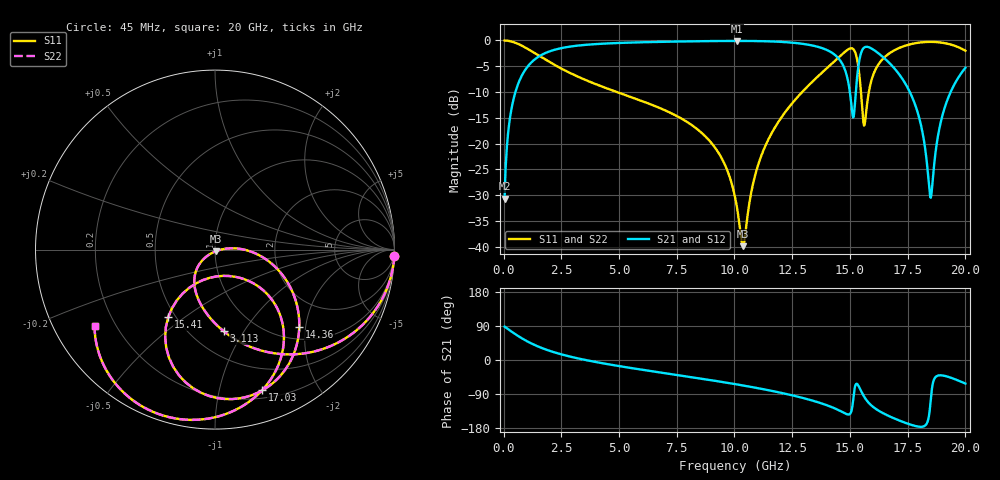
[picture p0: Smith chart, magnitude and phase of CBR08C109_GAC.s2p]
! S-parameter model data by Modelithics Inc.  support@modelithics.com 813-866-6335  Tampa FL USA
! S-Parameter data specifications:
! Substrate: 20-mil Rogers 4350B, substrate thickness, H=0.508mm, Dielectric constant, Er=3.75
! PCB Mounting Pad Footprint: Pad width, PadW=1.45mm , Pad length, PadL=1mm , Pad gap, PadG (edge-to-edge)=0.6mm , Reference planes=2.6mm apart
#  GHz  S  MA  R 50
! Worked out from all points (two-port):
!   801 points, 45 MHz to 20 GHz, reference 50 ohm
!   highest |S21| = -0.10 dB at 10.1 GHz (marker M1); lowest = -30.7 dB at 45 MHz (marker M2)
!   |S21| within 3 dB of the highest: 1.531 GHz to 14.42 GHz (12.89 GHz wide, 162 % of centre); 15.44 GHz to 16.4 GHz (958.7 MHz wide, 6.02 % of centre)
!   lowest |S11| = -39.9 dB at 10.37 GHz (marker M3), VSWR 1.02, Z = 50.4 - j0.946 ohm
!   |S11| at or under -10 dB: 4.911 GHz to 12.93 GHz (8.019 GHz wide, 89.9 % of centre); 15.48 GHz to 15.82 GHz (340.9 MHz wide, 2.18 % of centre)
!   |S22| runs from -39.9 to 0.0 dB; largest |S21 - S12| = 0
!   S11 on the Smith chart (normalised r, x): 45 MHz: 1, -58; 3.113 GHz: 0.71, -0.82; 14.36 GHz: 1.27, -1.85; 15.41 GHz: 0.46, -0.44; 17.03 GHz: 0.27, -1.35; 20 GHz: 0.12, -0.29
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0.045  0.9996 -2.0  0.02928 88.0  0.02928 88.0  0.9996 -2.0
0.319381  0.979 -14.0  0.2034 76.0  0.2034 76.0  0.979 -14.0
0.793312  0.8887 -32.7  0.4573 57.2  0.4573 57.2  0.8887 -32.7
3.113081  0.4572 -83.9  0.8857 5.7  0.8857 5.7  0.4572 -83.9
3.387462  0.4291 -87.5  0.8994 2.0  0.8994 2.0  0.4291 -87.5
6.704981  0.2243 -120.8  0.9681 -32.2  0.9681 -32.2  0.2243 -120.8
8.974863  0.1032 -138.8  0.9858 -53.2  0.9858 -53.2  0.1032 -138.8
10.0225  0.03046 -135.4  0.989 -63.6  0.989 -63.6  0.03046 -135.4
10.09733  0.02489 -131.5  0.989 -64.4  0.989 -64.4  0.02489 -131.5
10.37171  0.01017 -67.4  0.9888 -67.3  0.9888 -67.3  0.01017 -67.4
11.31958  0.0933 4.5  0.9822 -77.9  0.9822 -77.9  0.0933 4.5
13.36496  0.3969 -20.2  0.894 -106.9  0.894 -106.9  0.3969 -20.2
14.36271  0.638 -42.6  0.7207 -128.2  0.7207 -128.2  0.638 -42.6
15.13597  0.827 -89.2  0.1792 -107.6  0.1792 -107.6  0.827 -89.2
15.41035  0.4581 -124.7  0.6495 -72.6  0.6495 -72.6  0.4581 -124.7
15.63484  0.1531 -72.9  0.8586 -98.7  0.8586 -98.7  0.1531 -72.9
16.68248  0.7432 -62.2  0.6126 -147.8  0.6126 -147.8  0.7432 -62.2
17.03169  0.826 -71.4  0.5018 -157.1  0.5018 -157.1  0.826 -71.4
17.95461  0.9498 -94.7  0.1934 -175.7  0.1934 -175.7  0.9498 -94.7
18.50337  0.9686 -108.4  0.02996 -102.3  0.02996 -102.3  0.9686 -108.4
19.05214  0.9459 -122.3  0.2045 -41.3  0.2045 -41.3  0.9459 -122.3
20  0.7948 -147.6  0.5435 -62.2  0.5435 -62.2  0.7948 -147.6
